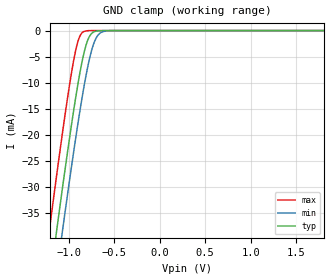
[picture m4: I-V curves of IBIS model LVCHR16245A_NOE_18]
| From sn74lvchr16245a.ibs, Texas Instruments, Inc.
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[Model]   LVCHR16245A_NOE_18
Model_type  Input
Vinl=0.5775
Vinh=1.2675
| variable   typ   min   max
C_comp   3.44pF   2.65pF   4.47pF
[Temperature Range]   40   100   -40
| Ambient temperature   25   85   -40
[Voltage range]   1.8   1.65   1.95
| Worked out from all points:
|   GND clamp passes 1 mA (typ) near -0.77 V on its own axis
[GND Clamp]
| LVCHR16245A_NOE_18
|   Voltage   I(typ)   I(min)   I(max)
-5.5V     -655.2mA   -662.2mA   -646.6mA
-1.215V   -49.6mA    -57.88mA   -38.96mA
-1.135V   -39.07mA   -47.36mA   -28.42mA
-1.075V   -31.35mA   -39.6mA    -20.75mA
-1.055V   -28.82mA   -37.05mA   -18.27mA
-955mV    -16.68mA   -24.66mA   -6.874mA
-885mV    -9.098mA   -16.55mA   -1.486mA
-825mV    -3.922mA   -10.26mA   -137.1uA
-780mV    -1.472mA   -6.227mA   -17.15uA
-715mV    -205.4uA   -2.128mA   -808.5nA
-650mV    -22.01uA   -443.9uA   -37.93nA
1.8V      3.326pA    6.142pA    3.026pA
